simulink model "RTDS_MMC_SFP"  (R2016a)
settings: Solver=FixedStepAuto  StartTime=0.0  StopTime=0.4  RelTol=1e-3
PreLoadFcn:
  | % --- DO NOT REMOVE THIS CODE (2024.3.b1) ---
  |     % create Simulink variants
  |     if not(exist('variant_simulation', 'var'))
  |         variant_simulation = Simulink.Variant('SIMULINK_MODE==0');
  |     end
  |     if not(exist('variant_generation', 'var'))
  |         variant_generation = Simulink.Variant('SIMULINK_MODE==1');
  |     end
  | 
  |     % check SDK version
  |     required_lib_version = 3900.3;
  |     required_lib_ver_str = '2024.3';
  |     lib_path = [getenv('IX_SIMULINK_ACG_BB_3') '\simulink\blocks\BoomBox.slx'];
  |     if exist(lib_path, 'file')
  |         lib_version = str2double(Simulink.MDLInfo(lib_path).ModelVersion); % fullpath to avoid getting shadowing files
  |         if lib_version < required_lib_version || isnan(lib_version)
  |             error(['The model ''' bdroot ''' has been saved with a more recent version of ACG SDK (' required_lib_ver_str ') and might not work as expected. <a href="matlab:private_end_string = ''--- PLACE YOUR CODE BELOW THIS LINE ---'';private_fcn = get_param(bdroot, ''PreLoadFcn'');private_end_index = strfind(private_fcn, private_end_string);set_param(bdroot, ''PreLoadFcn'', strtrim(private_fcn(private_end_index(end)+length(private_end_string):end)));private_fcn = get_param(bdroot, ''PostLoadFcn'');private_end_index = strfind(private_fcn, private_end_string);set_param(bdroot, ''PostLoadFcn'', strtrim(private_fcn(private_end_index(end)+length(private_end_string):end)));private_fcn = get_param(bdroot, ''InitFcn'');private_end_index = strfind(private_fcn, private_end_string);set_param(bdroot, ''InitFcn'', strtrim(private_fcn(private_end_index(end)+length(private_end_string):end)));clear private_end_string private_fcn private_end_index;open(bdroot);">Click here</a> to continue anyway, or download the latest version of the SDK at <a href="www.imperix.com/downloads">www.imperix.ch/downloads</a>.']);
  |         end
  |     elseif exist(getenv('IX_SIMULINK_ACG_BB_3'), 'dir')
  |         error(['Library file for imperix ACG SDK not found in path ''' lib_path '''. Please try to re-install ACG SDK (<a href="www.imperix.com/downloads">www.imperix.ch/downloads</a>).']);
  |     else
  |         error('ACG SDK is not installed on this computer and the model will not work as expected. Please download ACG SDK at <a href="www.imperix.com/downloads">www.imperix.ch/downloads</a>, install it, and reopen the model.');
  |     end
  |     clear required_lib_version required_lib_ver_str lib_path lib_version;
  | 
  |     ix_acg_path = getenv('IX_SIMULINK_ACG_BB_3');
  |     addpath(fullfile(ix_acg_path, 'simulink\target'));
  |     addpath(fullfile(ix_acg_path, 'simulink\blocks'));
  |     addpath(fullfile(ix_acg_path, 'simulink\functions'));
  |     sl_refresh_customizations;
  |     clear ix_acg_path;
  | 
  |     % The SIMULINK_MODE variable is created in the base
  |     % workspace in the PostLoadFcn from the block whose id is kb0101
  |     % All opened models share a common variant configuration.
  | 
  |     Model_PreLoadFcn(bdroot);
  | % --- PLACE YOUR CODE BELOW THIS LINE ---
PostLoadFcn:
  | % --- DO NOT REMOVE THIS CODE (2024.3.b1) ---
  |     % change the execution mode of simulink depending on the radio button:
  |     if(strcmp('Automated Code Generation',get_param(Find_imperix_blocks(bdroot,'Configuration'),'SLMODE')))
  |         assignin('base', 'SIMULINK_MODE', 1);
  |     else
  |         assignin('base', 'SIMULINK_MODE', 0);
  |     end
  | 
  |     Model_PostLoadFcn(bdroot);
  | % --- PLACE YOUR CODE BELOW THIS LINE ---
InitFcn:
  | % --- DO NOT REMOVE THIS CODE (2024.3.b1) ---
  |     % check SDK version
  |     required_lib_version = 3900.3;
  |     required_lib_ver_str = '2024.3';
  |     lib_path = [getenv('IX_SIMULINK_ACG_BB_3') '\simulink\blocks\BoomBox.slx'];
  |     if exist(lib_path, 'file')
  |         lib_version = str2double(Simulink.MDLInfo(lib_path).ModelVersion); % fullpath to avoid getting shadowing files
  |         if lib_version < required_lib_version || isnan(lib_version)
  |             error(['The model ''' bdroot ''' has been saved with a more recent version of ACG SDK (' required_lib_ver_str ') and might not work as expected. <a href="matlab:private_end_string = ''--- PLACE YOUR CODE BELOW THIS LINE ---'';private_fcn = get_param(bdroot, ''PreLoadFcn'');private_end_index = strfind(private_fcn, private_end_string);set_param(bdroot, ''PreLoadFcn'', strtrim(private_fcn(private_end_index(end)+length(private_end_string):end)));private_fcn = get_param(bdroot, ''PostLoadFcn'');private_end_index = strfind(private_fcn, private_end_string);set_param(bdroot, ''PostLoadFcn'', strtrim(private_fcn(private_end_index(end)+length(private_end_string):end)));private_fcn = get_param(bdroot, ''InitFcn'');private_end_index = strfind(private_fcn, private_end_string);set_param(bdroot, ''InitFcn'', strtrim(private_fcn(private_end_index(end)+length(private_end_string):end)));clear private_end_string private_fcn private_end_index;open(bdroot);">Click here</a> to continue anyway, or download the latest version of the SDK at <a href="www.imperix.com/downloads">www.imperix.ch/downloads</a>.']);
  |         end
  |     elseif exist(getenv('IX_SIMULINK_ACG_BB_3'), 'dir')
  |         error(['Library file for imperix ACG SDK not found in path ''' lib_path '''. Please try to re-install ACG SDK (<a href="www.imperix.com/downloads">www.imperix.ch/downloads</a>).']);
  |     else
  |         error('ACG SDK is not installed on this computer and the model will not work as expected. Please download ACG SDK at <a href="www.imperix.com/downloads">www.imperix.ch/downloads</a>, install it, and reopen the model.');
  |     end
  |     clear required_lib_version required_lib_ver_str lib_path lib_version;
  | 
  |     Model_InitFcn(bdroot);
  | % --- PLACE YOUR CODE BELOW THIS LINE ---
model workspace (MAT data in the model file):
  CTRLPERIOD = 0.0002
  TSAMPLE = 2e-06
  global_CLK_number = 0
  global_INT_number = 1
  global_SVM_instance_id = 0
  global_can_baud_rate = '1000000'
  global_comp_time = 0.2
  global_cycle_delay = 8e-05
  global_ip_addresses : cell (value not decoded)
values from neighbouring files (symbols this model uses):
  Ki_Vleg = 1/Ti    (= 2.95256991686)    [RTDS_MMC_SFP_init.m]
  Kp_Vleg = Tn/Ti    (= 0.14880952381)    [RTDS_MMC_SFP_init.m]
  N = 4    [RTDS_MMC_SFP_init.m]
  scale_factor = 0.5^16    (= 1.52587890625e-05)    [RTDS_MMC_SFP_init.m]
  Tsw = 1/fsw    (= 0.0008)    [RTDS_MMC_SFP_init.m]
  Vsm_max = 250    [RTDS_MMC_SFP_init.m]
undefined symbols (not defined in the file or in its folder): B, Board, Box, channel, DT, lane, Micro, ns, PRO, RCP, TPI, Vf
libraries: BoomBox x183, simulink x55
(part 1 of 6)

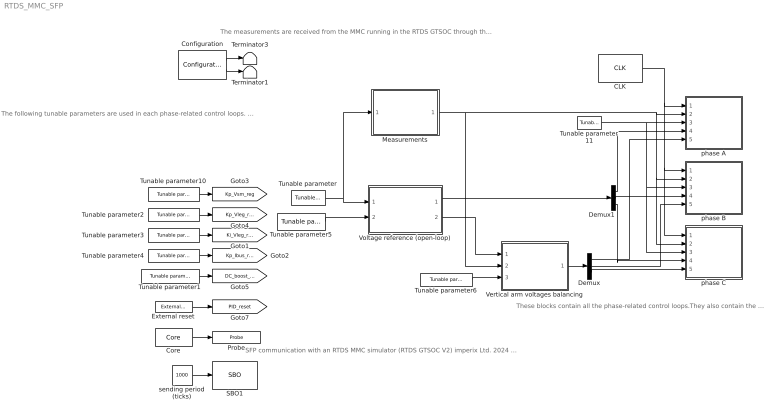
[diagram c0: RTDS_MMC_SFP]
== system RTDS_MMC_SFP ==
  note: SFP communication with an RTDS MMC simulator (RTDS GTSOC V2) imperix Ltd. 2024 Learn more about this example.
  note: The following tunable parameters are used in each phase-related control loops. The reset block allows to reset the integral part of each regulator when the pwm outputs are disabled.
  note: The measurements are received from the MMC running in the RTDS GTSOC through the SFP port.
  note: These blocks contain all the phase-related control loops.They also contain the configuration of the carrier-based pulse width modulators.
  CLK : BoomBox/CLK  CLK_ID=CLOCK_1  CLK_FREQ=fsw  VAR_FREQ=off  LIM_FREQ=[10e3 50e3]  KBID=kb0102
  Configuration : BoomBox/Configuration  Description=Please leave the Priority (below parameter) to maximum negative to ensure that this block is always executed first.  Priority=-99999  SLMODE=Automated Code Generation  load_from_file=on  init_file=RTDS_MMC_SFP_init.m  clk0_freq=fs  interrupt_phase=0  interrupt_pstsclr=0  clk0_is_variable=on  sampling_conf=Disabled  nb_oversamples=0  sampling_phases=[0.2 0.8]  adc_delay_conf=2000 ns (B-Box RCP, B-Box Micro, B-Board PRO or TPI)  custom_adc_delay=off  adc_delay_s=500e-9  Parameter15=0  MAXSTEP=auto  MINSTEP=auto  RELTOL=1e-3  TSAMPLE=1e-6  computation_time=0.4  cycle_delay_unit=Period  powerlib_model=(A) Simple  powerlib_switch=Switching devices (switched)  powerlib_pwm=PWM signals  KBID=kb0101  interrupt_presc_real=1  interrupt_ticks_real=50000  highest_device_id=0
  Core : BoomBox/Core  show_reset=off  KBID=kb0503
  Demux : Demux  Outputs=[1 1 1]
  Demux1 : Demux  Outputs=3
  External reset : BoomBox/External reset  KBID=kb0504
  Measurements : Subsystem
  Probe : BoomBox/Probe  VARNAME=core_state  EVALUATE=Literal  DATATYPE=single  CAN_ENABLED=off  CAN_ADDRESS=0  CAN_TX_FREQ=10  init_baudrate=0  CAN_BAUDRATE=1000000  can_endianness=Little-endian  ETH_ENABLED=off  ETH_PORT=2000  ETH_IP_LIST=IP address 0  eth_endianness=Little-endian  ETH_TX_FREQ=10  init_ip=0  KBID=kb0502  CAN_BIG_ENDIAN=0  ETH_BIG_ENDIAN=0  ETH_IP_SFCN=empty  CAN_MB_ID=0  ETH_MB_ID=1  RESIZE=0
  SBO1 : BoomBox/SBO  NB_BBX=0  START_REG_RT=00  NB_REG_RT=1  START_REG=00  NB_REG=0  VAL1=0  VAL2=0  VAL3=0  VAL4=0  VAL5=0  VAL6=0  VAL7=0  VAL8=0  KBID=kb0210
  Terminator1 : Terminator
  Terminator3 : Terminator
  Tunable parameter5 : BoomBox/Tunable parameter  VARNAME=M_inv  EVALUATE=Literal  INITIALVAL=0.3  DATA_TYPE=single  VAL_MAX=Inf  VAL_MIN=-Inf  CAN_ENABLED=off  CAN_ADDRESS=0  can_endianness=Little-endian  init_baudrate=0  CAN_BAUDRATE=1000000  ETH_ENABLED=off  ETH_PORT=2000  eth_endianness=Little-endian  SIM_OUT=Steps  STEP_TIMES=[0 0.2]  STEP_DATA=[0.2 0.3]  KBID=kb0501  CAN_BIG_ENDIAN=0  ETH_BIG_ENDIAN=0  CAN_MB_ID=0  ETH_MB_ID=1  RESIZE=0
  Tunable parameter : BoomBox/Tunable parameter  VARNAME=Vdc  EVALUATE=Literal  INITIALVAL=Vdc  DATA_TYPE=single  VAL_MAX=Inf  VAL_MIN=-Inf  CAN_ENABLED=off  CAN_ADDRESS=0  can_endianness=Little-endian  init_baudrate=0  CAN_BAUDRATE=1000000  ETH_ENABLED=off  ETH_PORT=2000  eth_endianness=Little-endian  SIM_OUT=Initial value  STEP_TIMES=[0.1 0.2]  STEP_DATA=[1 2]  KBID=kb0501  CAN_BIG_ENDIAN=0  ETH_BIG_ENDIAN=0  CAN_MB_ID=1  ETH_MB_ID=2  RESIZE=0
  Tunable parameter1 : BoomBox/Tunable parameter  VARNAME=DC_bus_ratio  EVALUATE=Literal  INITIALVAL=1.1  DATA_TYPE=single  VAL_MAX=Inf  VAL_MIN=-Inf  CAN_ENABLED=off  CAN_ADDRESS=0  can_endianness=Little-endian  init_baudrate=0  CAN_BAUDRATE=1000000  ETH_ENABLED=off  ETH_PORT=2000  eth_endianness=Little-endian  SIM_OUT=Steps  STEP_TIMES=[0 0.1]  STEP_DATA=[1.1 1.2]  KBID=kb0501  CAN_BIG_ENDIAN=0  ETH_BIG_ENDIAN=0  CAN_MB_ID=0  ETH_MB_ID=1  RESIZE=0
  Tunable parameter10 : BoomBox/Tunable parameter  VARNAME=Kp_Vsm_reg  EVALUATE=Literal  INITIALVAL=Kp_Vsm  DATA_TYPE=single  VAL_MAX=Inf  VAL_MIN=-Inf  CAN_ENABLED=off  CAN_ADDRESS=0  can_endianness=Little-endian  init_baudrate=0  CAN_BAUDRATE=1000000  ETH_ENABLED=off  ETH_PORT=2000  eth_endianness=Little-endian  SIM_OUT=Initial value  STEP_TIMES=[0.1 0.2]  STEP_DATA=[1 2]  KBID=kb0501  CAN_BIG_ENDIAN=0  ETH_BIG_ENDIAN=0  CAN_MB_ID=0  ETH_MB_ID=1  RESIZE=0
  Tunable parameter11 : BoomBox/Tunable parameter  VARNAME=Pff  EVALUATE=Literal  INITIALVAL=0  DATA_TYPE=single  VAL_MAX=Inf  VAL_MIN=-Inf  CAN_ENABLED=off  CAN_ADDRESS=0  can_endianness=Little-endian  init_baudrate=0  CAN_BAUDRATE=1000000  ETH_ENABLED=off  ETH_PORT=2000  eth_endianness=Little-endian  SIM_OUT=Initial value  STEP_TIMES=[0.1 0.2]  STEP_DATA=[1 2]  KBID=kb0501  CAN_BIG_ENDIAN=0  ETH_BIG_ENDIAN=0  CAN_MB_ID=0  ETH_MB_ID=1  RESIZE=0
  Tunable parameter2 : BoomBox/Tunable parameter  VARNAME=Kp_Vleg_reg  EVALUATE=Literal  INITIALVAL=Kp_Vleg  DATA_TYPE=single  VAL_MAX=Inf  VAL_MIN=-Inf  CAN_ENABLED=off  CAN_ADDRESS=0  can_endianness=Little-endian  init_baudrate=0  CAN_BAUDRATE=1000000  ETH_ENABLED=off  ETH_PORT=2000  eth_endianness=Little-endian  SIM_OUT=Initial value  STEP_TIMES=[0.1 0.2]  STEP_DATA=[1 2]  KBID=kb0501  CAN_BIG_ENDIAN=0  ETH_BIG_ENDIAN=0  CAN_MB_ID=0  ETH_MB_ID=1  RESIZE=0
  Tunable parameter3 : BoomBox/Tunable parameter  VARNAME=Ki_Vleg_reg  EVALUATE=Literal  INITIALVAL=Ki_Vleg  DATA_TYPE=single  VAL_MAX=Inf  VAL_MIN=-Inf  CAN_ENABLED=off  CAN_ADDRESS=0  can_endianness=Little-endian  init_baudrate=0  CAN_BAUDRATE=1000000  ETH_ENABLED=off  ETH_PORT=2000  eth_endianness=Little-endian  SIM_OUT=Initial value  STEP_TIMES=[0.1 0.2]  STEP_DATA=[1 2]  KBID=kb0501  CAN_BIG_ENDIAN=0  ETH_BIG_ENDIAN=0  CAN_MB_ID=0  ETH_MB_ID=1  RESIZE=0
  Tunable parameter4 : BoomBox/Tunable parameter  VARNAME=Kp_Ibus_reg  EVALUATE=Literal  INITIALVAL=Kp_Ibus  DATA_TYPE=single  VAL_MAX=Inf  VAL_MIN=-Inf  CAN_ENABLED=off  CAN_ADDRESS=0  can_endianness=Little-endian  init_baudrate=0  CAN_BAUDRATE=1000000  ETH_ENABLED=off  ETH_PORT=2000  eth_endianness=Little-endian  SIM_OUT=Initial value  STEP_TIMES=[0.1 0.2]  STEP_DATA=[1 2]  KBID=kb0501  CAN_BIG_ENDIAN=0  ETH_BIG_ENDIAN=0  CAN_MB_ID=0  ETH_MB_ID=1  RESIZE=0
  Tunable parameter6 : BoomBox/Tunable parameter  VARNAME=Kp_bal_reg  EVALUATE=Literal  INITIALVAL=0.1  DATA_TYPE=single  VAL_MAX=Inf  VAL_MIN=-Inf  CAN_ENABLED=off  CAN_ADDRESS=0  can_endianness=Little-endian  init_baudrate=0  CAN_BAUDRATE=1000000  ETH_ENABLED=off  ETH_PORT=2000  eth_endianness=Little-endian  SIM_OUT=Initial value  STEP_TIMES=[0.1 0.2]  STEP_DATA=[1 2]  KBID=kb0501  CAN_BIG_ENDIAN=0  ETH_BIG_ENDIAN=0  CAN_MB_ID=0  ETH_MB_ID=1  RESIZE=0
  Vertical arm voltages balancing : Subsystem
  Voltage reference (open-loop) : Subsystem
  phase A : Subsystem
  phase B : Subsystem
  phase C : Subsystem
  sending period (ticks) : Constant  Value=1000  OutDataTypeStr=uint16
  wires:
  Tunable parameter10/1 -> [Kp_Vsm_reg]
  External reset/1 -> [PID_reset]
  Measurements/1(acqdata) -> Vertical arm voltages balancing/2(acqdata), phase A/2(acqdata), phase C/2(acqdata), phase B/2(acqdata)
  Tunable parameter4/1 -> [Kp_Ibus_reg]
  Configuration/1 -> Terminator3/1
  Tunable parameter11/1 -> phase A/3(Pff), phase C/3(Pff), phase B/3(Pff)
  Demux1/2 -> phase B/4(Eac)
  Demux1/3 -> phase C/4(Eac)
  Demux1/1 -> phase A/4(Eac)
  CLK/1 -> phase A/1(PWM_CLK), phase B/1(PWM_CLK), phase C/1(PWM_CLK)
  Tunable parameter2/1 -> [Kp_Vleg_reg]
  Demux/2 -> phase B/5(I_bal)
  Vertical arm voltages balancing/1(Ibal_abc) -> Demux/1
  Tunable parameter6/1 -> Vertical arm voltages balancing/3(Kp_bal)
  Demux/3 -> phase C/5(I_bal)
  Tunable parameter1/1 -> [DC_boost_ratio]
  Voltage reference (open-loop)/1(Eabc_ref) -> Demux1/1
  Tunable parameter3/1 -> [Ki_Vleg_reg]
  Demux/1 -> phase A/5(I_bal)
  Tunable parameter5/1 -> Voltage reference (open-loop)/2(Vdc)
  Voltage reference (open-loop)/2(theta) -> Vertical arm voltages balancing/1(theta)
  Tunable parameter/1 -> Voltage reference (open-loop)/1(M_inv), Measurements/1(Vdc)
  Configuration/2 -> Terminator1/1
  Core/1 -> Probe/1
  sending period (ticks)/1 -> SBO1/1
